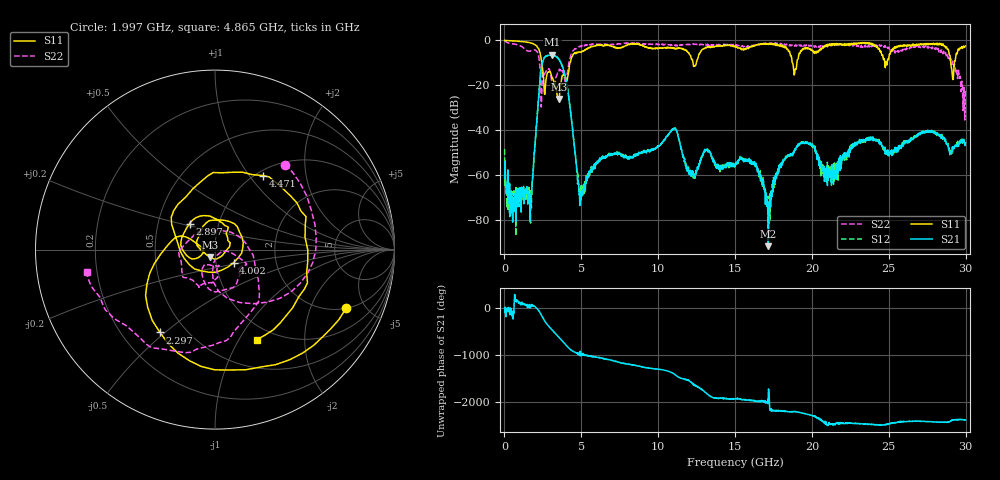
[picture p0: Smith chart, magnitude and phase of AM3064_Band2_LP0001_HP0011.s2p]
# Hz S DB R 50.0
!freq dBS11 angS11 dBS21 angS21 dBS12 angS12 dBS22 angS22
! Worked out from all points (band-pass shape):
!   1600 points, 10 MHz to 29.98 GHz, reference 50 ohm
!   highest |S21| = -6.40 dB at 3.103 GHz (marker M1); lowest = -91.6 dB at 17.16 GHz (marker M2)
!   |S21| within 3 dB of the highest: 2.49 GHz to 3.633 GHz (1.143 GHz wide, 37.3 % of centre)
!   lowest |S11| = -26.1 dB at 3.553 GHz (marker M3), VSWR 1.10, Z = 47.4 - j4.02 ohm
!   |S11| at or under -10 dB: 2.424 GHz to 4.266 GHz (1.842 GHz wide, 55.1 % of centre); 18.73 GHz to 19.02 GHz (290.2 MHz wide, 1.54 % of centre); 29.03 GHz to 29.26 GHz (230.5 MHz wide, 0.791 % of centre)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
!   |S22| runs from -35.4 to -0.2 dB; largest |S21 - S12| = 0.016
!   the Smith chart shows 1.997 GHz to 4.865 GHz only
!   S11 on the Smith chart (normalised r, x): 1.997 GHz: 2.02, -3.65; 2.297 GHz: 0.36, -0.48; 2.897 GHz: 0.72, +0.22; 4.002 GHz: 1.22, -0.18; 4.471 GHz: 1.07, +1.17; 4.865 GHz: 0.83, -1.20
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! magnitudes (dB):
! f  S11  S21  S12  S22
! 10 MHz  0.0  -61.2  -48.4  -0.2
! 291.2 MHz  -0.1  -72.8  -64.9  -1.2
! 1.622 GHz  -0.9  -68.9  -69.9  -4.8
! 1.997 GHz  -1.9  -45.5  -45.5  -4.2
! 2.297 GHz  -5.1  -18.8  -18.8  -11.0
! 2.897 GHz  -13.9  -6.6  -6.6  -12.6
! 3.103 GHz  -16.8  -6.4  -6.5  -19.4
! 3.553 GHz  -26.1  -8.7  -8.5  -13.3
! 4.002 GHz  -18.0  -17.5  -17.6  -18.6
! 4.471 GHz  -6.2  -42.4  -42.1  -4.5
! 4.865 GHz  -5.1  -68.9  -65.9  -2.8
! 5.015 GHz  -5.2  -67.0  -65.8  -2.7
! 10 GHz  -3.4  -47.1  -47.0  -1.7
! 15 GHz  -2.7  -55.5  -55.6  -1.9
! 16.28 GHz  -2.2  -55.1  -55.9  -2.2
! 17.16 GHz  -1.6  -91.6  -83.3  -1.4
! 18.17 GHz  -2.5  -53.5  -53.7  -2.1
! 19.99 GHz  -4.2  -46.4  -47.2  -2.1
! 21.13 GHz  -1.6  -58.1  -56.6  -2.5
! 25 GHz  -8.0  -50.9  -50.7  -3.0
! 28.56 GHz  -2.2  -43.5  -43.5  -4.8
! 29.98 GHz  -2.5  -45.7  -46.3  -21.8
